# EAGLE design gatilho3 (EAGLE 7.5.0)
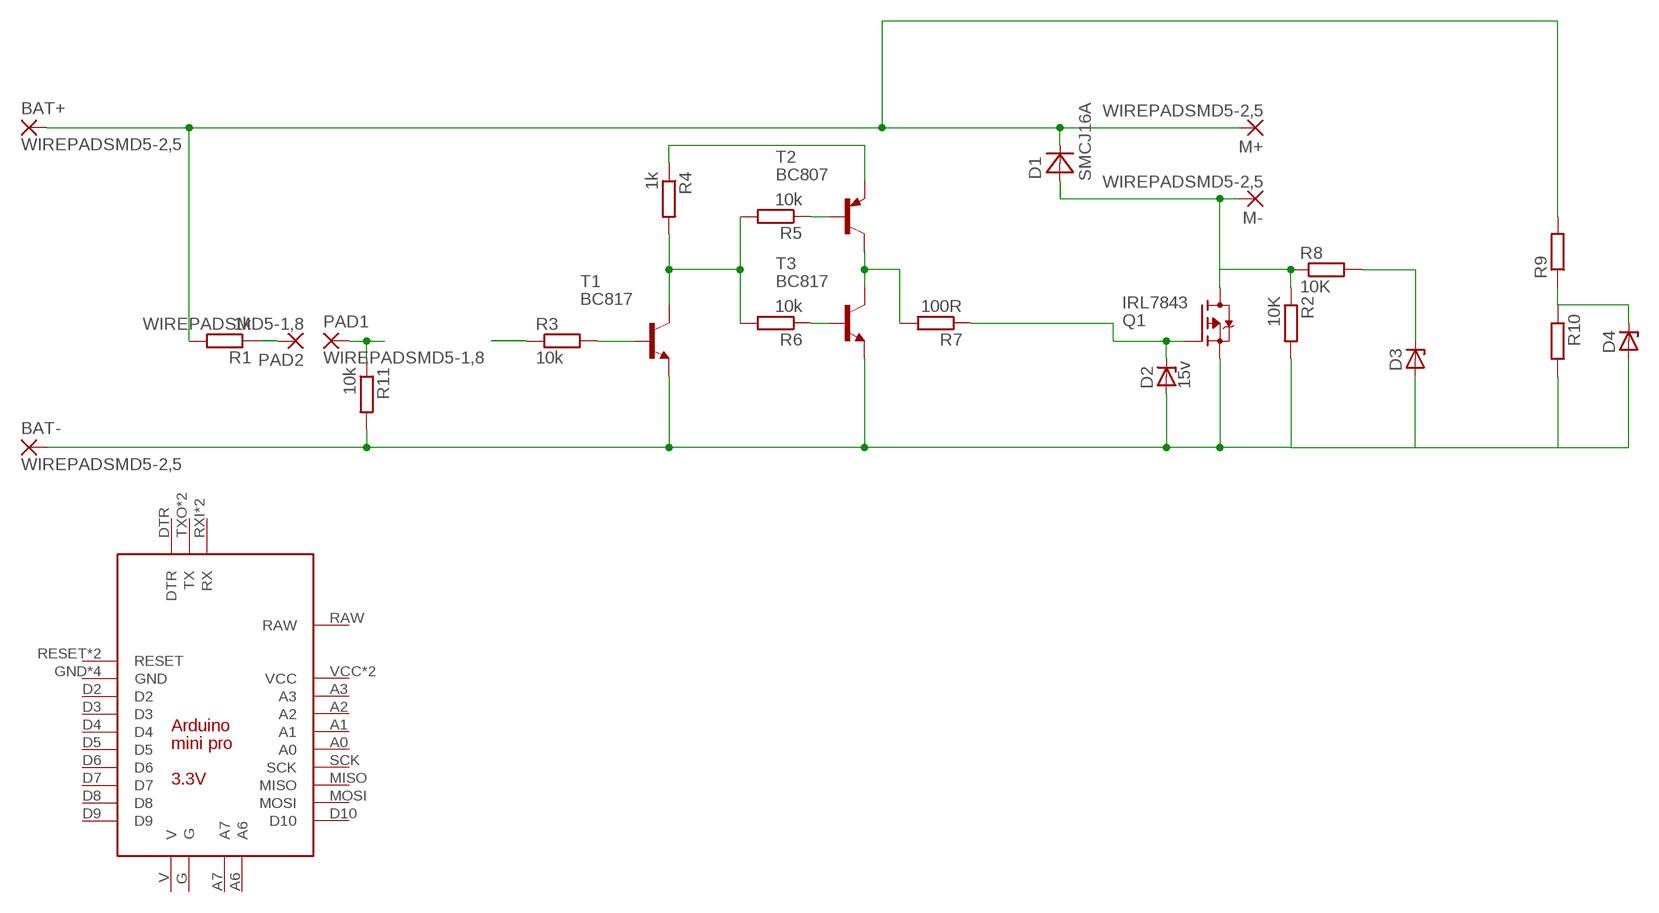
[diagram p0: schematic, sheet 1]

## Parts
BAT+  WIREPADSMD5-2,5  [5-2,5]
BAT-  WIREPADSMD5-2,5  [5-2,5]
D1  SMCJ16A  MBRA340T3  [SMA]
D2  15v  ZENER-DIODESOD80C  [SOD80C]
D3  ZENER-DIODESOD80C  [SOD80C]
D4  ZENER-DIODESOD80C  [SOD80C]
M+  WIREPADSMD5-2,5  [5-2,5]
M-  WIREPADSMD5-2,5  [5-2,5]
PAD1  WIREPADSMD5-1,8  [5-1,8]
PAD2  WIREPADSMD5-1,8  [5-1,8]
Q1  IRL7843  FDD4141TO252  [TO252]
R1  1k  R-EU_R0805  [R0805]
R2  10K  R-EU_R0805  [R0805]
R3  10k  R-EU_R0805  [R0805]
R4  1k  R-EU_R0805  [R0805]
R5  10k  R-EU_R0805  [R0805]
R6  10k  R-EU_R0805  [R0805]
R7  100R  R-EU_R0805  [R0805]
R8  10K  R-EU_R0805  [R0805]
R9  R-EU_R0805  [R0805]
R10  R-EU_R0805  [R0805]
R11  10k  R-EU_R0805  [R0805]
T1  BC817  MMBT3904LT1-NPN-SOT23-BEC  [SOT23-BEC]
T2  BC807  MMBT3906LT1-PNP-SOT23-BEC  [SOT23-BEC]
T3  BC817  MMBT3904LT1-NPN-SOT23-BEC  [SOT23-BEC]
U$1  ARDUINO_MINI_PRO_3V3  [ARDUINO_MINI_PRO_3V3]

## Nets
N$1: BAT-.1(P) D2.A D3.A D4.A Q1.2(S) R2.2 R10.2 R11.2 T1.E T3.E
N$2: D1.A M-.1(P) Q1.3(D) R2.1 R8.1
N$3: D4.C R9.1 R10.1
N$4: PAD2.1(P) R1.1
N$5: BAT+.1(P) D1.C M+.1(P) R1.2 R9.2
N$6: PAD1.1(P) R11.1
N$7: R3.1
N$8: D3.C R8.2
N$9: R4.1 T2.E
N$11: R4.2 R5.2 R6.2 T1.C
N$12: R3.2 T1.B
N$13: R7.2 T2.C T3.C
N$15: R5.1 T2.B
N$16: R6.1 T3.B
N$17: D2.C Q1.1(G) R7.1
Unconnected: U$1.A0 U$1.A1 U$1.A2 U$1.A3 U$1.A6 U$1.A7 U$1.D2 U$1.D3 U$1.D4 U$1.D5 U$1.D6 U$1.D7 U$1.D8 U$1.D9 U$1.D10 U$1.DTR U$1.G U$1.GND U$1.GND2(GND) U$1.GND3(GND) U$1.GND4(GND) U$1.MISO U$1.MOSI U$1.RAW U$1.RESET U$1.RESET2(RESET) U$1.RXI2(RX) U$1.RXI(RX) U$1.SCK U$1.TXO2(TX) U$1.TXO(TX) U$1.V U$1.VCC U$1.VCC2(VCC)

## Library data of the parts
BAT+ BAT- M+ M- PAD1 PAD2 = wirepad:WIREPAD: Wire PAD connect wire on PCB
D1 = diode:MBRA340T3: Surface Mount Schottky Power Rectifier
D2-D4 = diode:ZENER-DIODE: Z-Diode
Q1 = transistor-fet:FDD4141: P-Channel PowerTrench® MOSFET Source: FDD4141.pdf
R1-R11 = resistor:R-EU_: RESISTOR, European symbol
T1 T3 = transistor-neu-to92:*-NPN-: NPN Transistror
T2 = transistor:*-PNP-: PNP Transistror
U$1 = eBay parts:ARDUINO_MINI_PRO_3V3: 3.3 V Arduino pro module from eBay NOTE: Untested layout; ARDUINO: 3.3V

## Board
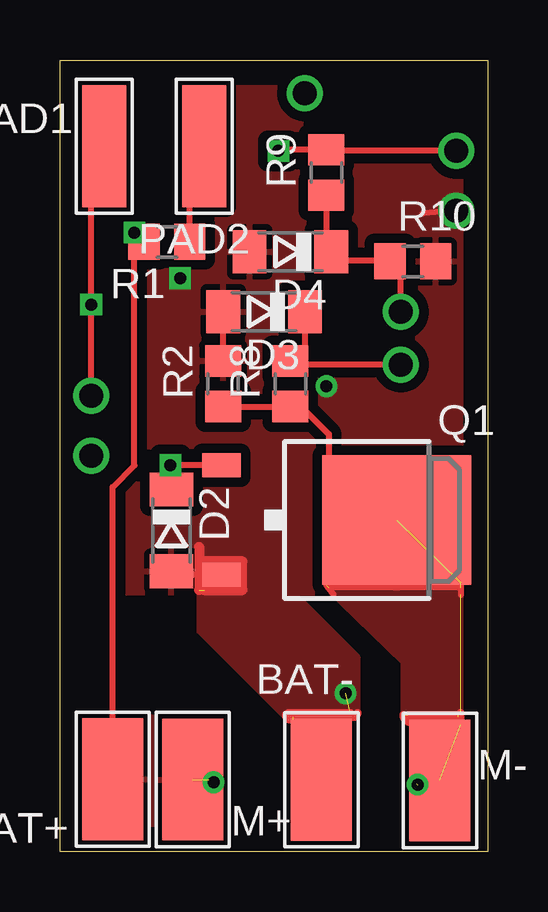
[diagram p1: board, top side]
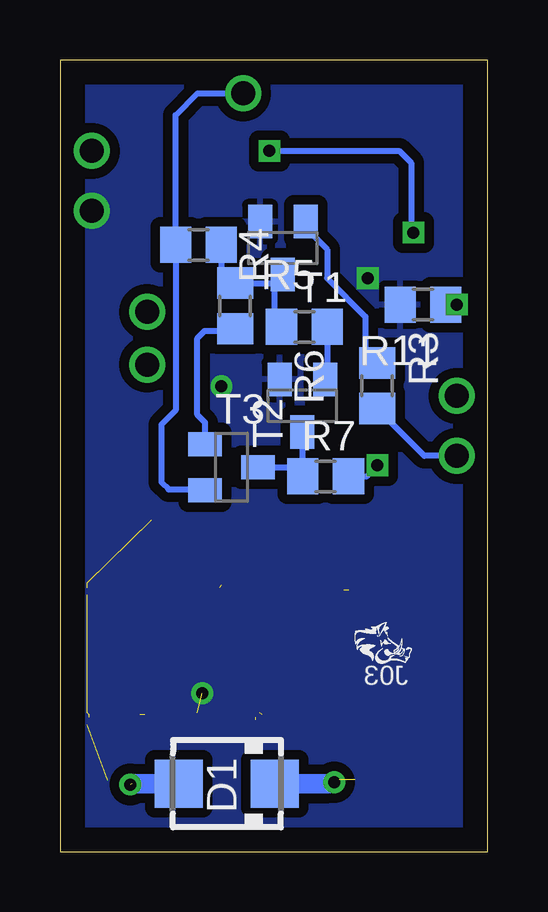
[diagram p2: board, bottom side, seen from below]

Size 17.83 x 32.99 mm. Coordinates in mm from the lower left corner, seen from the top.
Outline: 17.82,32.99 0,32.99 0,0 17.82,0
Outline: 17.83,32.99 17.83,0
Copper layers (1*16): Top 0.035mm / dielectric 1.5mm / Bottom 0.035mm
Design rules "default": minimum track width 10mil, minimum drill 24mil, track to track 8mil, track to pad 8mil, pad to pad 8mil, via to via 8mil, smd to smd 8mil, copper to edge 40mil, drill to drill 8mil, minimum pad ring 10mil, minimum via ring 8mil, stop-mask expansion 4mil, vias tented up to drill 0mil, thermal gap 10mil

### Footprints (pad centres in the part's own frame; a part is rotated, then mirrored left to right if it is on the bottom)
5-2,5 = smd 2.54 x 5.08: 1 0,0
SMA = smd 2 x 2: A 2,0; C -2,0
SOD80C = smd 1.4 x 1.8: A 1.7,0; C -1.7,0
5-1,8 = smd 1.829 x 5.08: 1 0,0
TO252 = smd 1 x 1.6: 1 -2.28,-4.8; 2 2.28,-4.8 | smd 5.4 x 6.2: 3 0,2.5
R0805 = smd 1.3 x 1.5: 1 -0.95,0; 2 0.95,0
SOT23-BEC = smd 1 x 1.4: B -0.95,-1.1; C 0,1.1; E 0.95,-1.1
ARDUINO_MINI_PRO_3V3 = drill 1.016 pad 1.88: A0 7.62,-5.08; A1 7.62,-2.54; A2 7.62,0; A3 7.62,2.54; A6 5.08,-15.24; A7 2.54,-15.24; D2 -7.62,2.54; D3 -7.62,0; D4 -7.62,-2.54; D5 -7.62,-5.08; D6 -7.62,-7.62; D7 -7.62,-10.16; D8 -7.62,-12.7; D9 -7.62,-15.24; D10 7.62,-15.24; DTR 6.35,15.24; G -2.54,-15.24; GND -7.62,5.08; GND2 7.62,10.16; GND3 -6.35,15.24; GND4 -3.81,15.24; MISO 7.62,-10.16; MOSI 7.62,-12.7; RAW 7.62,12.7; RESET -7.62,7.62; RESET2 7.62,7.62; RXI -7.62,10.16; RXI2 1.27,15.24; SCK 7.62,-7.62; TXO -7.62,12.7; TXO2 3.81,15.24; V -5.08,-15.24; VCC 7.62,5.08; VCC2 -1.27,15.24

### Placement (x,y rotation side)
BAT+  2.19,3.03 180 top
BAT-  10.89,3 0 top
D1  10.87,2.84 180 bottom
D2  4.65,13.39 270 top
D3  8.5,22.5 180 top
D4  9.6,25 180 top
M+  5.53,3.01 180 top
M-  15.83,2.97 0 top
PAD1  1.85,29.4 180 top
PAD2  6,29.4 0 top
Q1  11.53,13.82 270 top
R1  4.45,25.41 180 top
R2  6.8,19.5 90 top
R3  4.61,19.42 90 bottom
R4  12.05,25.29 0 bottom
R5  10.53,22.75 90 bottom
R6  7.65,21.88 180 bottom
R7  6.76,15.64 180 bottom
R8  9.6,19.5 90 top
R9  11.1,28.3 90 top
R10  14.7,24.6 0 top
R11  2.7,22.8 180 bottom
T1  8.54,25.15 180 bottom
T2  10.68,16.02 270 bottom
T3  7.73,18.58 180 bottom
U$1  not placed on the board

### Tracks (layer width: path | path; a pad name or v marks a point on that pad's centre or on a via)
N$1  (via drill 0.5, 1)  (4 unrouted)
  Top 0.254: Q1.2 4.39,11.54 D2.A | R2.2 D3.A | v16.5,26.7 15.1,26.6
  Top 0.305: 9.7,5.6 12.2,5.6 arc90 12.4,5.8 | 12.1,5.8 9.5,5.8 | 9.7,5.5 9.6,5.5 arc-90 9.4,5.7
  Top 0.406: 6,10.9 7.6,10.9 7.6,12.1 6,12.1 | 5.8,12.7 5.8,10.9
  Top 1.27: BAT-.1
  other vias: 11.9,6.6 11.1,19.4 5,23.9
  pour Bottom (isolate 0.406): 0.1,33 17.8,33 17.8,0.1 0.1,0.1
  pour Top: 12.4,5.6 12.4,8.1 8.4,12.1 6,12.1 5.8,11.9 5.8,9.2 9.5,5.5 12.3,5.5
  pour Top (isolate 0.406): 0,33 17.9,33 17.9,10.8 0,10.8
N$2  (via drill 0.5)  (9 unrouted)
  Top 0.254: R2.1 R8.1 10.05,18.55 11.2,17.4 11.2,16.3 11.5,16 11.85,16 Q1.3 | v14.9,2.8 15.66,2.8 M-.1 | 16.7,11 11.2,11 | 11.1,11.1 11.4,10.7 | 16.7,11.2 16.7,10.7
  Top 0.305: 16.6,5.6 14.5,5.6 | 14.5,5.7 16.6,5.7 | 16.7,5.3 16.7,5.8 | 14.6,5.4 arc-90 14.3,5.7
  Bottom 0.813: D1.A 14.84,2.84
  pour Top: 11,11.1 11.1,11 14.3,7.9 14.3,5.7 14.6,5.4 17,5.4 17.2,5.6 17.2,11 17.1,11.1
N$3  (via drill 1)
  Top 0.254: 14.2,24.55 R10.1 | R9.1 11.1,25.2 D4.C 11.65,24.65 13.7,24.65 R10.1 | v14.2,22.5 14.2,24.15 R10.1
N$4
  Top 0.254: R1.1 5.4,28.8 PAD2.1
N$5  (via drill 0.5, 1)  (1 unrouted)
  Top 0.254: BAT+.1 2.19,15.2 3.1,16.1 v3.1,25.8 3.1,25.2 R1.2 | v16.5,29.2 11.15,29.2 R9.2 9.15,29.25 v9.1,29.2
  Top 0.406: v6.4,2.9 6.2,3
  Bottom 0.254: v9.1,29.2 3.7,29.2 3.2,28.7 3.2,25.8 v3.1,25.8
  Bottom 0.406: 6.64,2.84 v6.4,2.9
  Bottom 0.813: D1.C 6.64,2.84
  pour Top: 3.3,5.6 4.4,5.6 4.4,0.5 3.4,0.5 3.4,5.5
N$6  (via drill 0.5, 1)
  Top 0.254: v1.3,19 v1.3,22.8 1.3,28.85 PAD1.1
  Bottom 0.254: R11.1 v1.3,22.8
N$7  (via drill 1)
  Bottom 0.254: v1.3,16.5 2.64,16.5 R3.1
N$8  (via drill 1)
  Top 0.254: D3.C 10.2,20.25 R8.2 9.85,20.3 v14.2,20.3
N$9  (via drill 1)
  Bottom 0.254: T2.E 11.81,15.1 13.3,15.1 13.6,15.4 13.6,17.8 13.01,18.39 R4.1 13.01,30.7 12.1,31.6 v10.2,31.6
N$11
  Bottom 0.254: R5.2 8.9,23.7 | 8.9,23.7 T1.C | R5.2 10.53,23.62 10.5,23.59 | R4.2 11.11,24.27 R5.2 | 8.9,23.7 8.9,22.18 R6.2
N$12
  Bottom 0.254: T1.B 7.59,25.99 6.7,25.1 6.7,23.9 5.1,22.3 5.1,20.86 R3.2
N$13
  Bottom 0.254: T2.C 8.09,16.02 R7.2 7.73,15.66 T3.C
N$15
  Bottom 0.254: T2.B 11.78,17.88 12.1,18.2 12.1,21.4 11.8,21.7 10.62,21.7 R5.1
N$16
  Bottom 0.254: R6.1 6.7,19.77 T3.B
N$17  (via drill 0.5)
  Top 0.254: Q1.1 v4.6,16.1 4.64,16.05 D2.C 4.6,15.13
  Bottom 0.254: R7.1 5.05,15.64 v4.6,16.1

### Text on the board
bPlace: J03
